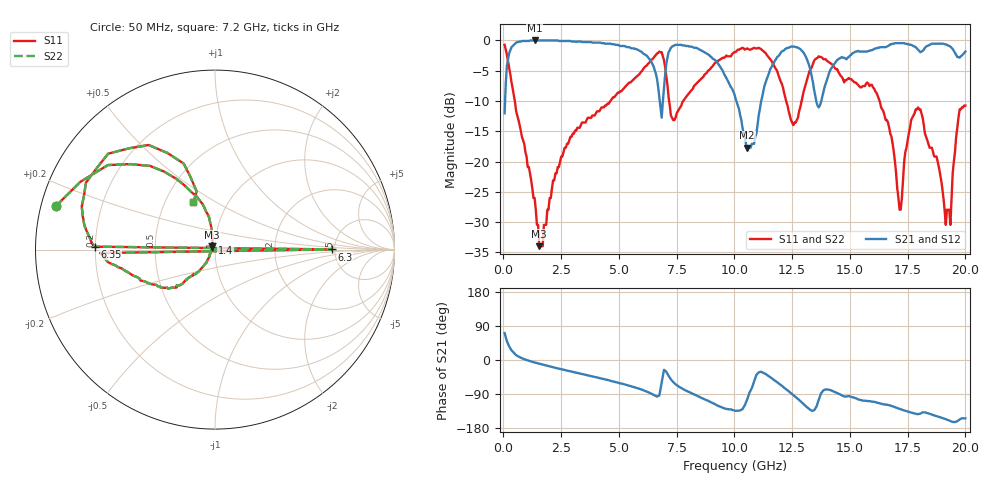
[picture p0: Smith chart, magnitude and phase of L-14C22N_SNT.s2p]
#	mhz	s	ma	r	50
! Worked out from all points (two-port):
!   400 points, 50 MHz to 20 GHz, reference 50 ohm
!   highest |S21| = 0.00 dB at 1.35 GHz (marker M1); lowest = -17.7 dB at 10.55 GHz (marker M2)
!   |S21| within 3 dB of the highest: 204.7 MHz to 6.305 GHz (6.1 GHz wide, 187 % of centre); 14.87 GHz to end of sweep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
!   lowest |S11| = -34.0 dB at 1.55 GHz (marker M3), VSWR 1.04, Z = 48.5 + j1.21 ohm
!   |S11| at or under -10 dB: 491.8 MHz to 4.631 GHz (4.14 GHz wide, 162 % of centre); 12.24 GHz to 12.91 GHz (671.5 MHz wide, 5.34 % of centre); 16.28 GHz to end of sweep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
!   |S22| runs from -34.0 to -0.7 dB; largest |S21 - S12| = 0
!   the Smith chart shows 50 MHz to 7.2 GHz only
!   S11 on the Smith chart (normalised r, x): 50 MHz: 0.04, +0.13; 1.4 GHz: 0.97, +0.07; 6.3 GHz: 4.71, +0.02; 6.35 GHz: 0.20, +0.01; 7.2 GHz: 0.69, +0.40
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50  0.92 164.8  0.25 71.1  0.25 71.1  0.92 164.8
500  0.31 108.8  0.94 15.9  0.94 15.9  0.31 108.8
1350  0.05 106.9  1 -6.6  1 -6.6  0.05 106.9
1400  0.04 113.4  1 -7.5  1 -7.5  0.04 113.4
1550  0.02 141.2  1 -10.0  1 -10.0  0.02 141.2
3400  0.21 -132.5  0.97 -36.9  0.97 -36.9  0.21 -132.5
6250  0.64 -178.3  0.73 -84.5  0.73 -84.5  0.64 -178.3
6300  0.65 0.1  0.71 -85.8  0.71 -85.8  0.65 0.1
6350  0.67 178.6  0.69 -87.2  0.69 -87.2  0.67 178.6
6700  0.79 157.4  0.41 -95.1  0.41 -95.1  0.79 157.4
7200  0.29 114.4  0.83 -46.4  0.83 -46.4  0.29 114.4
8350  0.44 160.3  0.87 -93.5  0.87 -93.5  0.44 160.3
10050  0.8 123.3  0.33 -134.2  0.33 -134.2  0.8 123.3
10550  0.86 106.6  0.13 -104.4  0.13 -104.4  0.86 106.6
12450  0.22 61.0  0.89 -87.7  0.89 -87.7  0.22 61.0
13350  0.6 94.3  0.5 -134.1  0.5 -134.1  0.6 94.3
14200  0.64 19.4  0.59 -80.5  0.59 -80.5  0.64 19.4
16700  0.19 -29.5  0.91 -119.3  0.91 -119.3  0.19 -29.5
17200  0.04 22.4  0.95 -130.1  0.95 -130.1  0.04 22.4
18050  0.27 49.0  0.8 -141.4  0.8 -141.4  0.27 49.0
19350  0.03 35.8  0.89 -160.9  0.89 -160.9  0.03 35.8
20000  0.29 -51.8  0.81 -154.1  0.81 -154.1  0.29 -51.8
